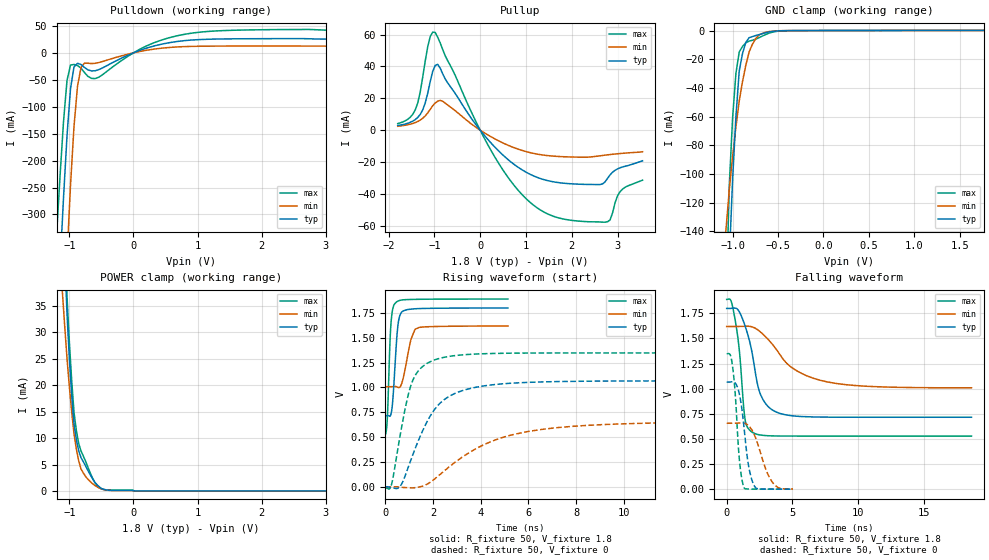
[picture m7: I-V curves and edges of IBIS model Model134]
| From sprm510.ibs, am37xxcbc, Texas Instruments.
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| Model based on original model for DSIPHY_WIO_ADDON_GPIOWRAPPER
|   Sub model FBPB_HS10L00_PD1_1P8
[model]   Model134
|[Input Load]   PD
|[Output Drive] SC10LB00
|Voltage   1.8V
|Mode   I/O
Model_type   I/O
Polarity   Non-Inverting
Enable   Active-Low
Vinl =  0.63
Vinh =  1.17
Cref =  15pF
Rref =  100.0000M
Vref =  0V
Vmeas =  0.9
C_comp   1.429432p   1.270657p   1.602015p
[Model Spec]
Vinl   0.63   0.567   0.6615
Vinh   1.17   1.053   1.2285
[Temperature Range]   25   125   -40
[Voltage Range]   1.8   1.62   1.89
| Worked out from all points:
|   slope of the pulldown table from 0 to 0.27 V, typ, clamps not added: 24.3 ohm
|   slope of the pullup table from 0 to 0.27 V, typ, clamps not added: 29.7 ohm
|   GND clamp passes 1 mA (typ) near -0.60 V on its own axis
|   POWER clamp passes 1 mA (typ) near -0.55 V on its own axis
|   rising waveform, R_fixture 50, V_fixture 1.8: 20-80 % time 179ps typ, 310ps min, 127ps max; typ from 0.715 V to 1.8 V
|   rising waveform, R_fixture 50, V_fixture 0: 20-80 % time 1.36ns typ, 3ns min, 720ps max; typ from 0 V to 1.06 V
|   falling waveform, R_fixture 50, V_fixture 1.8: 20-80 % time 1.1ns typ, 2.94ns min, 576ps max; typ from 1.8 V to 0.716 V
|   falling waveform, R_fixture 50, V_fixture 0: 20-80 % time 599ps typ, 1.04ns min, 415ps max; typ from 1.06 V to 0 V
[POWER_clamp]
-1.8V     362.5mA    191.4mA    412.8mA
-1.109V   56.74mA    37.73mA    60.49mA
-1.073V   44.66mA    31.25mA    47.92mA
-1.036V   33.51mA    25.07mA    36.71mA
-1V       25.05mA    19.75mA    28.19mA
-963.6mV  18.1mA     14.99mA    20.91mA
-927.3mV  12.67mA    10.8mA     14.87mA
-890.9mV  9.735mA    7.937mA    11.45mA
-818.2mV  6.3mA      4.158mA    7.553mA
-563.6mV  1.102mA    739.7uA    992.8uA
18.18mV   0A         0A         0A
3.6V      0A         0A         0A
[Pulldown]
-1.8V     -1.718A    -2.61A     -1.406A
-1.2V     -527.4mA   -844.5mA   -339.9mA
-1.145V   -396mA     -683.1mA   -229.1mA
-1.091V   -269mA     -526.7mA   -127.5mA
-1.036V   -153.6mA   -378.9mA   -51.17mA
-981.8mV  -66.33mA   -245.6mA   -22.67mA
-927.3mV  -26mA      -136.2mA   -21.54mA
-872.7mV  -19.34mA   -61.98mA   -23.69mA
-763.6mV  -27.2mA    -19.05mA   -36.72mA
-545.5mV  -31.39mA   -18.17mA   -45.46mA
872.7mV   23.46mA    11.88mA    35.92mA
3.545V    25.34mA    12.51mA    41.58mA
[Pullup]
-1.8V     2.903mA    2.423mA    4.112mA
-1.418V   6.595mA    4.711mA    12.64mA
-1.255V   12.69mA    7.42mA     33.24mA
-1.091V   30.4mA     13mA       58.69mA
-981.8mV  40.63mA    17.02mA    61.3mA
-818.2mV  35.38mA    18.12mA    50.59mA
272.7mV   -9.18mA    -4.728mA   -14.55mA
1.255V    -29.75mA   -15.09mA   -48.97mA
2.564V    -34.17mA   -16.31mA   -57.57mA
2.782V    -30.25mA   -15.5mA    -57.49mA
3.055V    -23.63mA   -14.68mA   -38.61mA
3.545V    -19.25mA   -13.56mA   -31.41mA
[GND_clamp]
-1.8V     -2.82A     -1.192A    -3.165A
-1.073V   -235.8mA   -138.4mA   -192.1mA
-1.036V   -159.6mA   -110.8mA   -107.6mA
-1V       -103.8mA   -87.86mA   -60.71mA
-963.6mV  -60.04mA   -67.29mA   -29.85mA
-927.3mV  -28.26mA   -49.1mA    -14.96mA
-890.9mV  -15.95mA   -35.5mA    -11.07mA
-854.5mV  -8.194mA   -24.09mA   -8.535mA
-818.2mV  -4.986mA   -14.87mA   -7.361mA
-709.1mV  -2.849mA   -3.094mA   -4.979mA
-563.6mV  -632.2uA   -437.1uA   -1.183mA
1.764V    97.78uA    55.01uA    156.3uA
[Ramp]
dV/dt_f  0.6516878/1.105603n   0.3685575/2.970803n   0.8181076/0.5773911n
dV/dt_r  0.6499197/1.366n   0.3999954/3.026171n   0.8218103/0.7214782n
R_load = 50
[Rising Waveform]
R_fixture = 50
V_fixture = 1.8
V_fixture_min = 1.62
V_fixture_max = 1.89
0s        715.2mV    1.007V     527.3mV
81ps      716.9mV    1.007V     709.3mV
180ps     709.8mV    1.007V     1.4V
234ps     734.5mV    1.007V     1.653V
297ps     844.7mV    1.007V     1.78V
396ps     1.204V     1.009V     1.843V
522ps     1.623V     1V         1.867V
729ps     1.766V     1.078V     1.88V
1.242ns   1.79V      1.584V     1.885V
5.139ns   1.798V     1.617V     1.888V
[Rising Waveform]
R_fixture = 50
V_fixture = 0
V_fixture_min = 0
V_fixture_max = 0
0s        -201.7uV   102.7uV    -10.06mV
243ps     -8.729mV   -231.3uV   13.72mV
666ps     23.47mV    -4.159mV   585.1mV
954ps     196mV      -8.598mV   923.6mV
1.143ns   320.2mV    -10.45mV   1.068V
1.557ns   562.3mV    7.434mV    1.209V
2.259ns   833.6mV    118.3mV    1.291V
4.266ns   1.019V     438.3mV    1.339V
6.588ns   1.055V     578.5mV    1.346V
20.58ns   1.065V     654.4mV    1.346V
[Falling Waveform]
R_fixture = 50
V_fixture = 1.8
V_fixture_min = 1.62
V_fixture_max = 1.89
0s        1.798V     1.619V     1.888V
324ps     1.799V     1.619V     1.876V
756ps     1.797V     1.618V     1.594V
1.422ns   1.616V     1.621V     675.6mV
2.007ns   1.303V     1.611V     561.5mV
2.394ns   1.017V     1.582V     543.3mV
2.763ns   891mV      1.542V     535.5mV
4.149ns   750.2mV    1.321V     528.7mV
8.145ns   716.2mV    1.056V     528.2mV
18.64ns   715.5mV    1.009V     528.2mV
[Falling Waveform]
R_fixture = 50
V_fixture = 0
V_fixture_min = 0
V_fixture_max = 0
0s        1.065V     656mV      1.346V
279ps     1.066V     656.1mV    1.334V
441ps     1.069V     656mV      1.228V
648ps     1.056V     656.1mV    953.7mV
972ps     941.3mV    658.7mV    285mV
1.323ns   610.6mV    657.7mV    15.25mV
1.683ns   220.5mV    629.9mV    1.597mV
2.133ns   25.68mV    532.5mV    275.4uV
3.492ns   362.5uV    67.22mV    8.168uV
5.04ns    66.46uV    1.641mV    961.7nV
